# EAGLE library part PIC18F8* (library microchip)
PIC18F87J10 FAMILY 64/80-Pin, High-Performance, 1-Mbit Flash Microcontrollers with nanoWatt Technology Source: http://www.microchip.com/ .. 39663c.pdf
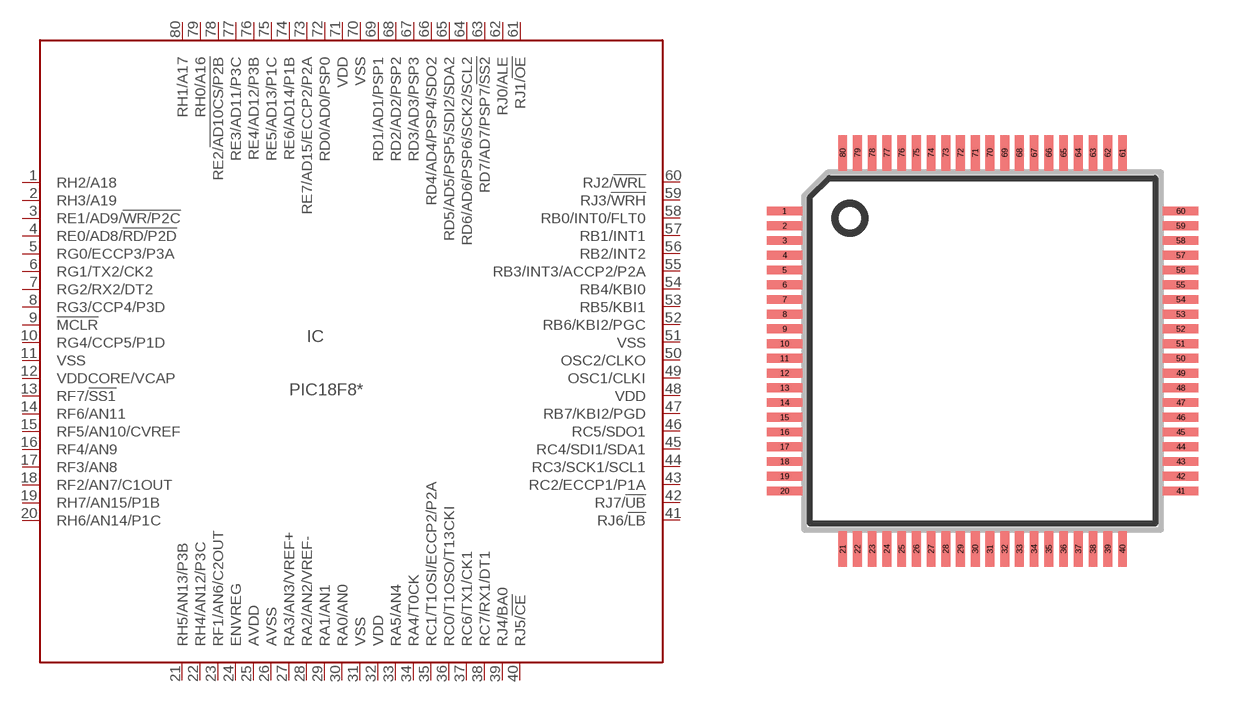
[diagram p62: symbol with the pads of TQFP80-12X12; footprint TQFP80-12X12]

Designator prefix IC

## PIC18F85J10 (MF: MICROCHIP; MPN: PIC18F85J10-I/PT; OC_FARNELL: 1847396; OC_NEWARK: 71J7277), PIC18F85J15 (MF: MICROCHIP; MPN: PIC18F85J15-I/PT; OC_FARNELL: unknown; OC_NEWARK: 71J7279), PIC18F86J10 (MPN: PIC18F86J10-I/PT; OC_FARNELL: 1332288; OC_NEWARK: 34M8058), PIC18F86J15 (MF: MICROCHIP; MPN: PIC18F86J15-I/PT; OC_FARNELL: unknown; OC_NEWARK: 71J7284), PIC18F87J10 (MF: MICROCHIP; MPN: PIC18F87J10-I/PT; OC_FARNELL: 1332290; OC_NEWARK: 71J7289)  [TQFP80-12X12]
1  RH2/A18
2  RH3/A19
3  RE1/AD9/!WR/P2C
4  RE0/AD8/!RD/P2D
5  RG0/ECCP3/P3A
6  RG1/TX2/CK2
7  RG2/RX2/DT2
8  RG3/CCP4/P3D
9  !MCLR  in
10  RG4/CCP5/P1D
11  VSS  pwr
12  VDDCORE/VCAP  pwr
13  RF7/!SS1
14  RF6/AN11
15  RF5/AN10/CVREF
16  RF4/AN9
17  RF3/AN8
18  RF2/AN7/C1OUT
19  RH7/AN15/P1B
20  RH6/AN14/P1C
21  RH5/AN13/P3B
22  RH4/AN12/P3C
23  RF1/AN6/C2OUT
24  ENVREG  in
25  AVDD  pwr
26  AVSS  pwr
27  RA3/AN3/VREF+
28  RA2/AN2/VREF-
29  RA1/AN1
30  RA0/AN0
31  VSS  pwr
32  VDD  pwr
33  RA5/AN4
34  RA4/T0CK
35  RC1/T1OSI/ECCP2/P2A
36  RC0/T1OSO/T13CKI
37  RC6/TX1/CK1
38  RC7/RX1/DT1
39  RJ4/BA0
40  RJ5/!CE
41  RJ6/!LB
42  RJ7/!UB
43  RC2/ECCP1/P1A
44  RC3/SCK1/SCL1
45  RC4/SDI1/SDA1
46  RC5/SDO1
47  RB7/KBI2/PGD
48  VDD  pwr
49  OSC1/CLKI  in
50  OSC2/CLKO  out
51  VSS  pwr
52  RB6/KBI2/PGC
53  RB5/KBI1
54  RB4/KBI0
55  RB3/INT3/ACCP2/P2A
56  RB2/INT2
57  RB1/INT1
58  RB0/INT0/FLT0
59  RJ3/!WRH
60  RJ2/!WRL
61  RJ1/!OE
62  RJ0/ALE
63  RD7/AD7/PSP7/!SS2
64  RD6/AD6/PSP6/SCK2/SCL2
65  RD5/AD5/PSP5/SDI2/SDA2
66  RD4/AD4/PSP4/SDO2
67  RD3/AD3/PSP3
68  RD2/AD2/PSP2
69  RD1/AD1/PSP1
70  VSS  pwr
71  VDD  pwr
72  RD0/AD0/PSP0
73  RE7/AD15/ECCP2/P2A
74  RE6/AD14/P1B
75  RE5/AD13/P1C
76  RE4/AD12/P3B
77  RE3/AD11/P3C
78  RE2/!AD10CS/P2B
79  RH0/A16
80  RH1/A17

## Footprint TQFP80-12X12 (pad centres in mm)
TQFP80 12x12x1 mm Body Source: http://www.microchip.com/ .. 39663c.pdf
smd 1.2 x 0.3: 1 -6.725,4.75; 2 -6.725,4.25; 3 -6.725,3.75; 4 -6.725,3.25; 5 -6.725,2.75; 6 -6.725,2.25; 7 -6.725,1.75; 8 -6.725,1.25; 9 -6.725,0.75; 10 -6.725,0.25; 11 -6.725,-0.25; 12 -6.725,-0.75; 13 -6.725,-1.25; 14 -6.725,-1.75; 15 -6.725,-2.25; 16 -6.725,-2.75; 17 -6.725,-3.25; 18 -6.725,-3.75; 19 -6.725,-4.25; 20 -6.725,-4.75; 41 6.725,-4.75; 42 6.725,-4.25; 43 6.725,-3.75; 44 6.725,-3.25; 45 6.725,-2.75; 46 6.725,-2.25; 47 6.725,-1.75; 48 6.725,-1.25; 49 6.725,-0.75; 50 6.725,-0.25; 51 6.725,0.25; 52 6.725,0.75; 53 6.725,1.25; 54 6.725,1.75; 55 6.725,2.25; 56 6.725,2.75; 57 6.725,3.25; 58 6.725,3.75; 59 6.725,4.25; 60 6.725,4.75
smd 0.3 x 1.2: 21 -4.75,-6.725; 22 -4.25,-6.725; 23 -3.75,-6.725; 24 -3.25,-6.725; 25 -2.75,-6.725; 26 -2.25,-6.725; 27 -1.75,-6.725; 28 -1.25,-6.725; 29 -0.75,-6.725; 30 -0.25,-6.725; 31 0.25,-6.725; 32 0.75,-6.725; 33 1.25,-6.725; 34 1.75,-6.725; 35 2.25,-6.725; 36 2.75,-6.725; 37 3.25,-6.725; 38 3.75,-6.725; 39 4.25,-6.725; 40 4.75,-6.725; 61 4.75,6.725; 62 4.25,6.725; 63 3.75,6.725; 64 3.25,6.725; 65 2.75,6.725; 66 2.25,6.725; 67 1.75,6.725; 68 1.25,6.725; 69 0.75,6.725; 70 0.25,6.725; 71 -0.25,6.725; 72 -0.75,6.725; 73 -1.25,6.725; 74 -1.75,6.725; 75 -2.25,6.725; 76 -2.75,6.725; 77 -3.25,6.725; 78 -3.75,6.725; 79 -4.25,6.725; 80 -4.75,6.725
